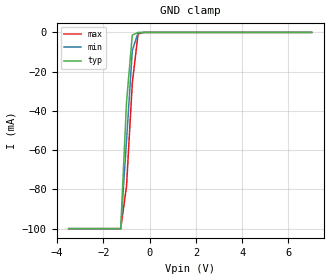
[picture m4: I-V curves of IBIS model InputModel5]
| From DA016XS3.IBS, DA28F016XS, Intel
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|**********************Input Model 5***************************************
[Model]   InputModel5
Model_type   Input
|   for CLK, ADV#
Vinl = 0.8V
Vinh = 2.0V
| Variable   typ   min   max
C_comp   5.61p   NA   7.6p
[Voltage Range]   3.3V   3.0V   3.6V
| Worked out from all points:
|   GND clamp passes 1 mA (typ) near -0.68 V on its own axis
[GND_clamp]
|Voltage I(typ)   I(min)   I(max)
-3.5V     -99.93mA   -99.94mA   -99.95mA
-1.25V    -99.93mA   -99.94mA   -99.95mA
-1V       -35.6mA    -55.38mA   -78.33mA
-750mV    -1.354mA   -9.196mA   -25.75mA
-500mV    -43.88uA   -197.8uA   -758.3uA
-250mV    0A         0A         -31.8uA
0V        0A         0A         0A
7V        0A         0A         0A
[POWER_clamp]
| Input buffer circuits of this product do not intrinsically
| require a [POWER_clamp] definition.  This zero current
| [POWER_clamp] is provided for compatibility with some ibis
| parsers.
|   Voltage  I(typ)   I(min)   I(max)
-3.3V     0A         0A         0A
-3V       0A         0A         0A
6.3V      0A         0A         0A
6.6V      0A         0A         0A
